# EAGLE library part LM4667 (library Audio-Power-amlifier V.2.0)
LM4667 Filterless High Efficiency 1.3W Switching Audio Amplifier
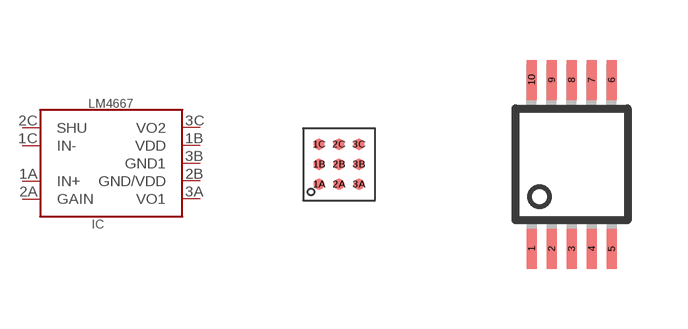
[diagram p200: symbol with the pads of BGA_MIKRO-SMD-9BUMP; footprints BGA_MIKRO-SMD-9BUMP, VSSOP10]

Designator prefix IC

## LM4667  [BGA_MIKRO-SMD-9BUMP]
1A  IN+  in
1B  VDD  pwr
1C  IN-  in
2A  GAIN
2B  GND/VDD  pwr
2C  SHU
3A  VO1  out
3B  GND1  pwr
3C  VO2  out

## LM4667LM4667MM  [VSSOP10]
1  SHU
2  IN-  in
4  IN+  in
5  GAIN
6  VO1  out
7  GND/VDD  pwr
8  GND1  pwr
9  VDD  pwr
10  VO2  out

## Footprint BGA_MIKRO-SMD-9BUMP (pad centres in mm)
BGA-Package Number TLA09 www.national.com
smd 0.277 x 0.277: 1A -0.5,-0.5; 1B -0.5,0; 1C -0.5,0.5; 2A 0,-0.5; 2B 0,0; 2C 0,0.5; 3A 0.5,-0.5; 3B 0.5,0; 3C 0.5,0.5

## Footprint VSSOP10 (pad centres in mm)
VSSOP10- DGS_(SPDSO-G10) www.ti.com/audio
smd 0.25 x 1: 1 -1,-2.113; 2 -0.5,-2.113; 3 0,-2.113; 4 0.5,-2.113; 5 1,-2.113; 6 1,2.113; 7 0.5,2.113; 8 0,2.113; 9 -0.5,2.113; 10 -1,2.113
